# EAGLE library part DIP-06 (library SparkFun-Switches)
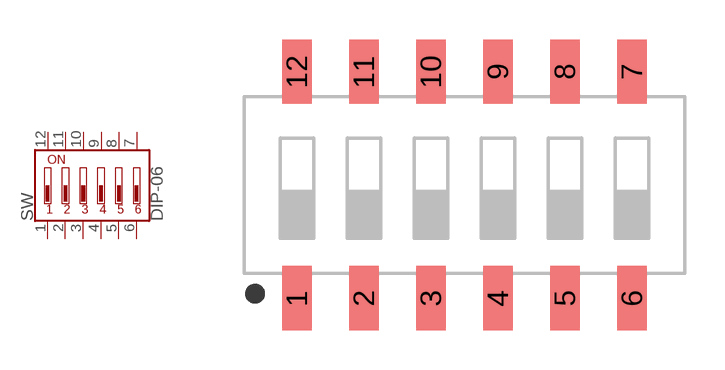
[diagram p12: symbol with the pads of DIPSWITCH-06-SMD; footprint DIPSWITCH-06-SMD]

Designator prefix SW

## DIP-06 (PROD_ID: --------)  [DIPSWITCH-06-SMD]
1  1
2  2
3  3
4  4
5  5
6  6
7  7
8  8
9  9
10  10
11  11
12  12

## Footprint DIPSWITCH-06-SMD (pad centres in mm)
smd 1.13 x 2.44: 1 -6.35,-4.3; 2 -3.81,-4.3; 3 -1.27,-4.3; 4 1.27,-4.3; 5 3.81,-4.3; 6 6.35,-4.3; 7 6.35,4.3; 8 3.81,4.3; 9 1.27,4.3; 10 -1.27,4.3; 11 -3.81,4.3; 12 -6.35,4.3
